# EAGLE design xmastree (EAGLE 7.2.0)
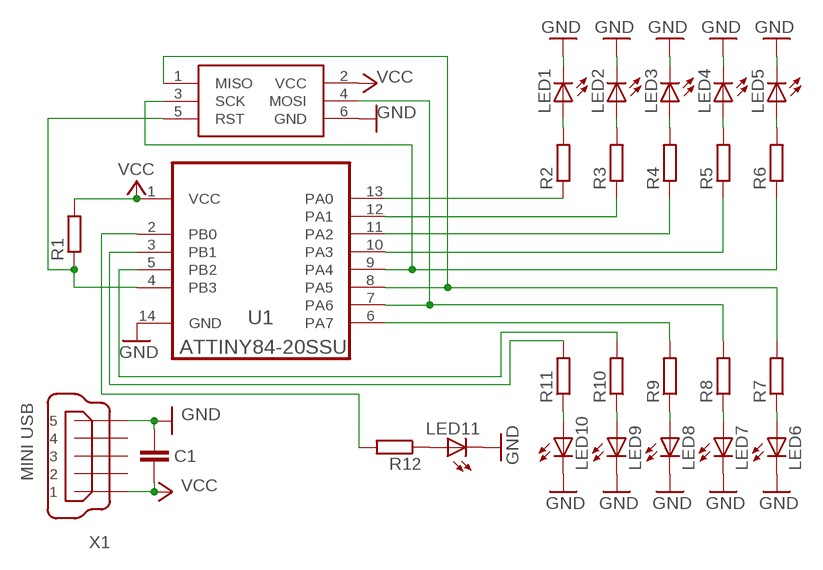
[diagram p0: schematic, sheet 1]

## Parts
C1  100nf  C-EUC1206  [C1206]
ISP1  AVRISP-6  [AVRISP]
LED1  LED3MM  [LED3MM]
LED2  LED3MM  [LED3MM]
LED3  LED3MM  [LED3MM]
LED4  LED3MM  [LED3MM]
LED5  LED3MM  [LED3MM]
LED6  LED3MM  [LED3MM]
LED7  LED3MM  [LED3MM]
LED8  LED3MM  [LED3MM]
LED9  LED3MM  [LED3MM]
LED10  LED3MM  [LED3MM]
LED11  LED5MM  [LED5MM]
R1  R-EU_R1206  [R1206]
R2  R-EU_R1206  [R1206]
R3  R-EU_R1206  [R1206]
R4  R-EU_R1206  [R1206]
R5  R-EU_R1206  [R1206]
R6  R-EU_R1206  [R1206]
R7  R-EU_R1206  [R1206]
R8  R-EU_R1206  [R1206]
R9  R-EU_R1206  [R1206]
R10  R-EU_R1206  [R1206]
R11  R-EU_R1206  [R1206]
R12  R-EU_R1206  [R1206]
U1  ATTINY84-20SSU  [SOIC127P600X175-14N]
X1  MINI USB  MINI-USB_SHIELD5P4-32005-400  [32005-400]

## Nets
GND: C1.1 ISP1.6(GND) LED1.K(C) LED2.K(C) LED3.K(C) LED4.K(C) LED5.K(C) LED6.K(C) LED7.K(C) LED8.K(C) LED9.K(C) LED10.K(C) LED11.K(C) U1.14(GND) X1.5
N$1: LED10.A R11.1
N$2: ISP1.5(RST) R1.1 U1.4(PB3)
N$3: LED7.A R8.1
N$4: LED8.A R9.1
N$5: ISP1.1(MISO) R7.2 U1.8(PA5)
N$6: ISP1.4(MOSI) R8.2 U1.7(PA6)
N$7: ISP1.3(SCK) R6.1 U1.9(PA4)
N$8: LED9.A R10.1
N$9: LED6.A R7.1
N$10: LED1.A R2.2
N$11: LED2.A R3.2
N$12: LED3.A R4.2
N$13: LED4.A R5.2
N$14: LED5.A R6.2
N$15: R12.2 U1.2(PB0)
N$16: R2.1 U1.13(PA0)
N$17: R3.1 U1.12(PA1)
N$18: R5.1 U1.10(PA3)
N$19: R4.1 U1.11(PA2)
N$21: R9.2 U1.6(PA7)
N$22: R10.2 U1.5(PB2)
N$23: R11.2 U1.3(PB1)
N$24: LED11.A R12.1
VCC: C1.2 ISP1.2(VCC) R1.2 U1.1(VCC) X1.1
Unconnected: X1.2 X1.3 X1.4 X1.M1(S1) X1.M2(S2) X1.M3(S3) X1.M4(S4)

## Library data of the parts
C1 = rcl:C-EU: CAPACITOR, European symbol
ISP1 = adafruit:AVRISP: AVR ISP HEADER Standard 6 pin header for AVR programming
LED1-LED11 = adafruit:LED: LED
R1-R12 = rcl:R-EU_: RESISTOR, European symbol
U1 = Atmel_By_element14_Batch_1-00:ATTINY84-20SSU: 8-bit Microcontroller with Bytes In-System Programmable Flash; MPN: ATTINY84-20SSU; OC_FARNELL: 1636955; OC_NEWARK: 03P2040; PACKAGE: SOIC-14; SUPPLIER: Atmel
X1 = con-cypressindustries:MINI-USB_SHIELD5P4-: MINI USB-B R/A W/O POST 5 pol. Source: www.cypressindustries.com; OC_FARNELL: unknown; OC_NEWARK: unknown

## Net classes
0 default: clearance 0.205 mm

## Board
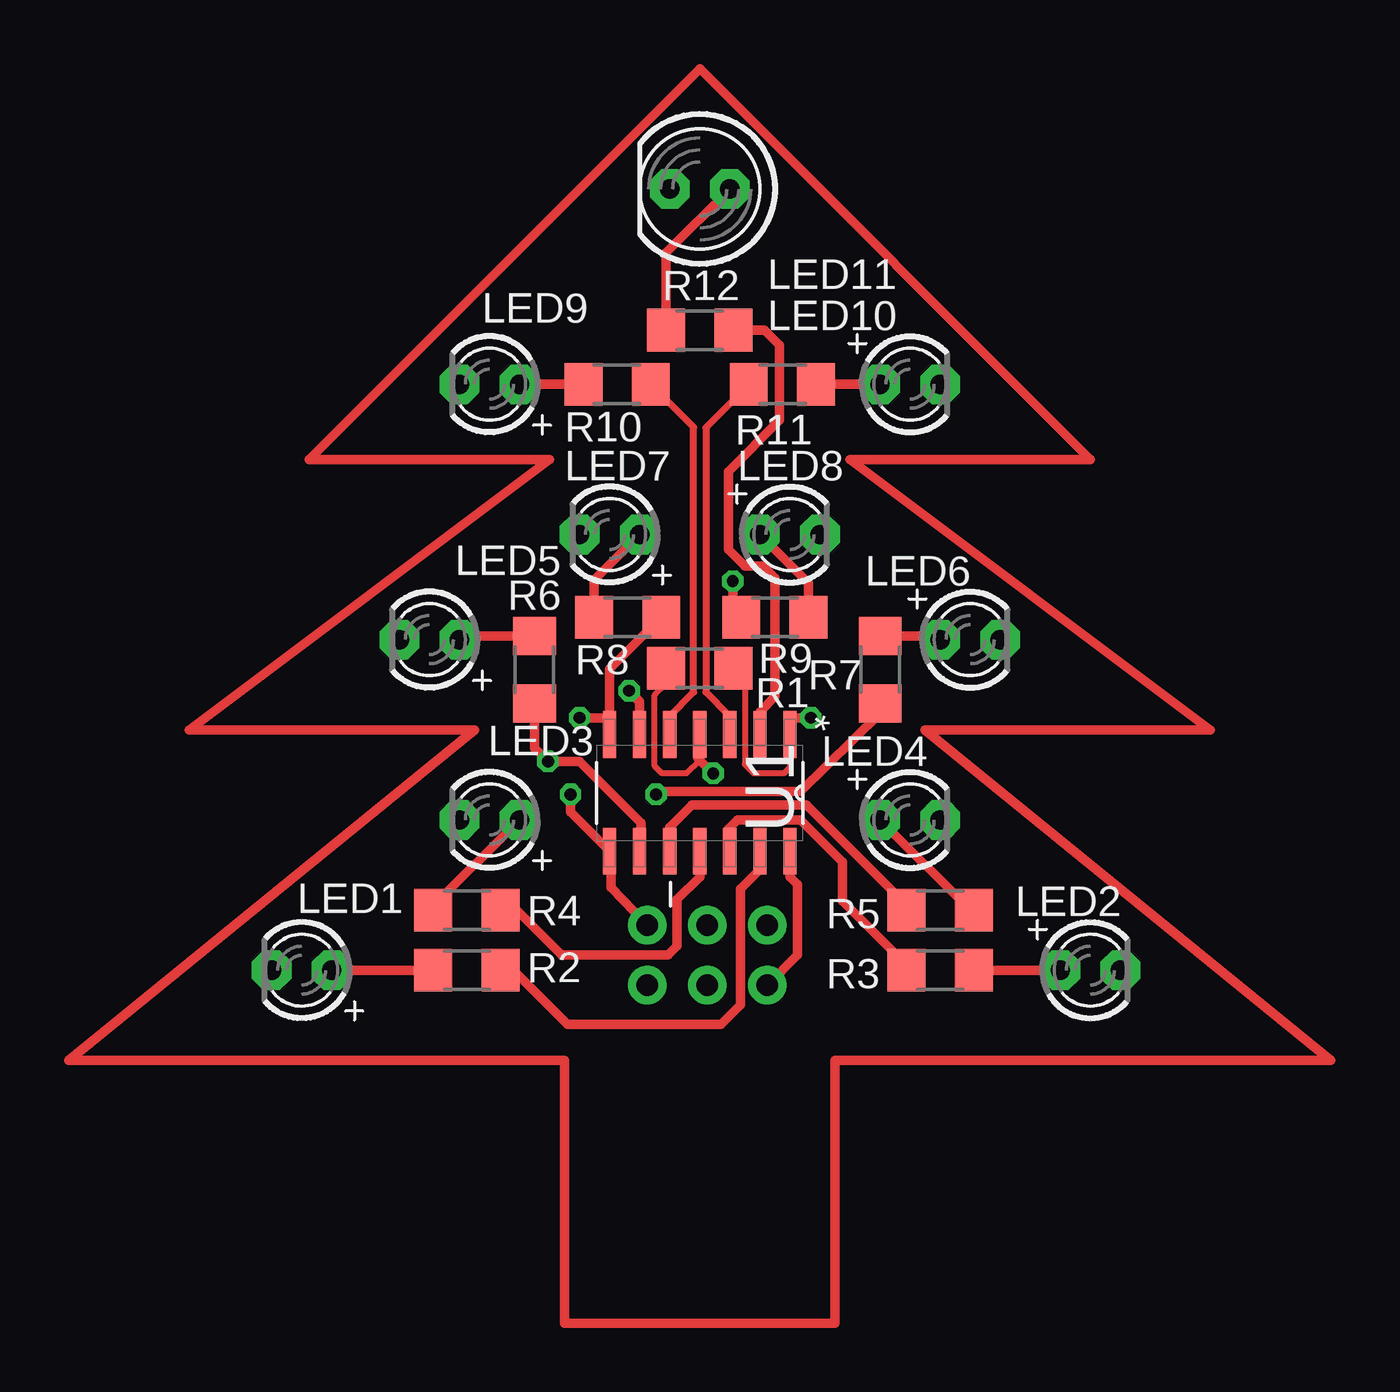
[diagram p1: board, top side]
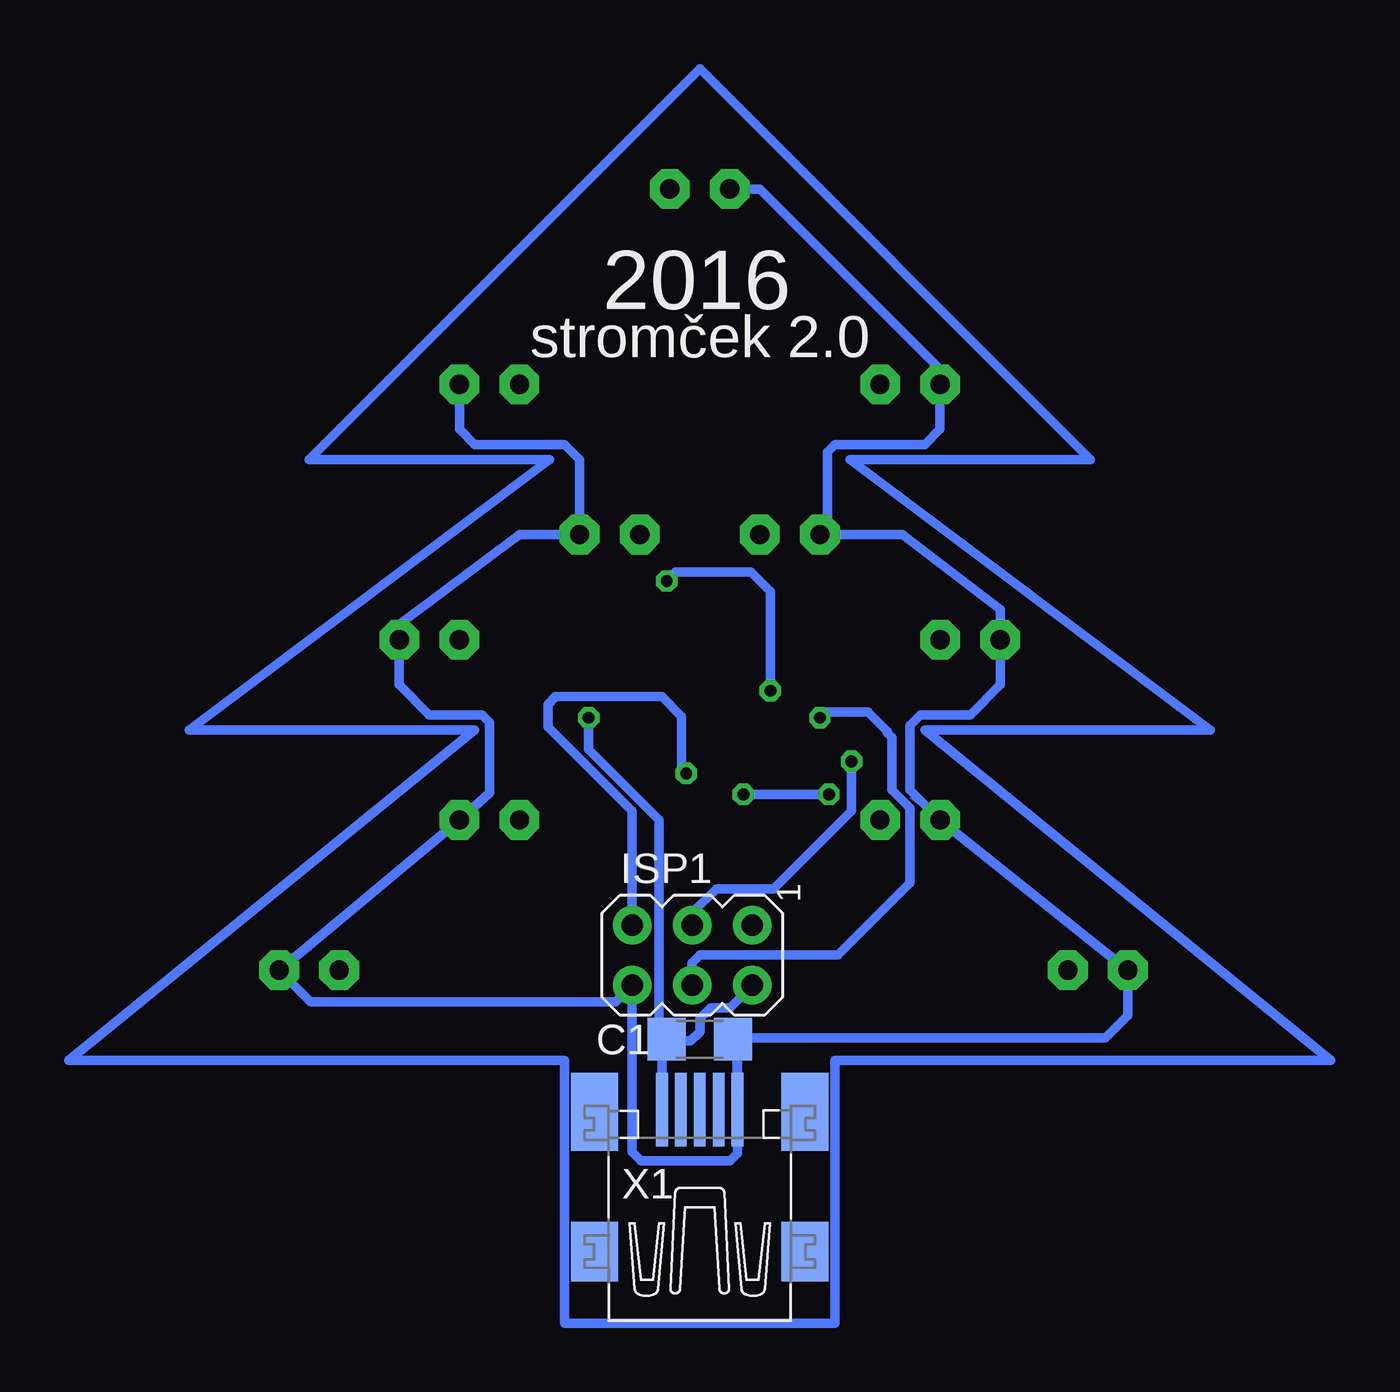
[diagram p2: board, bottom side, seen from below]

No outline drawn. Coordinates in mm, seen from the top.
Copper layers (1*16): Top 0.035mm / dielectric 1.5mm / Bottom 0.035mm
Design rules "default *": minimum track width 12mil, minimum drill 24mil, track to track 8mil, track to pad 8mil, pad to pad 8mil, via to via 8mil, smd to smd 8mil, copper to edge 40mil, drill to drill 8mil, minimum pad ring 10mil, minimum via ring 8mil, stop-mask expansion 4mil, vias tented up to drill 0mil, thermal gap 10mil

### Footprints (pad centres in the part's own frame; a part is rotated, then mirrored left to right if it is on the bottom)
C1206 = smd 1.6 x 1.8: 1 -1.4,0; 2 1.4,0
AVRISP = drill 0.9 pad 1.626: 1 -1.27,2.54; 2 1.27,2.54; 3 -1.27,0; 4 1.27,0; 5 -1.27,-2.54; 6 1.27,-2.54
LED3MM = drill 0.813 pad 1.676 octagon: A -1.27,0; K 1.27,0
LED5MM = drill 0.813 pad 1.676 octagon: A -1.27,0; K 1.27,0
R1206 = smd 1.6 x 1.803: 1 -1.422,0; 2 1.422,0
SOIC127P600X175-14N = smd 1.981 x 0.559: 1 -2.464,3.81; 2 -2.464,2.54; 3 -2.464,1.27; 4 -2.464,0; 5 -2.464,-1.27; 6 -2.464,-2.54; 7 -2.464,-3.81; 8 2.464,-3.81; 9 2.464,-2.54; 10 2.464,-1.27; 11 2.464,0; 12 2.464,1.27; 13 2.464,2.54; 14 2.464,3.81
32005-400 = smd 3.1 x 0.5: 1 3,1.6; 2 3,0.8; 3 3,0; 4 3,-0.8; 5 3,-1.6 | smd 2.5 x 2: M1 -3,-4.45; M2 -3,4.45 | smd 3.3 x 2: M3 2.9,4.45; M4 2.9,-4.45

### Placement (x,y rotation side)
C1  29.4,16.07 180 bottom
ISP1  29.72,19.62 270 bottom
LED1  12.57,18.99 180 top
LED2  45.91,18.99 0 top
LED3  20.51,25.34 180 top
LED4  38.29,25.34 0 top
LED5  17.97,32.96 180 top
LED6  40.83,32.96 0 top
LED7  25.59,37.4 180 top
LED8  33.21,37.4 0 top
LED9  20.51,43.75 180 top
LED10  38.29,43.75 0 top
LED11  29.4,52.01 180 top
R1  29.4,31.75 0 top
R2  19.56,18.99 180 top
R3  39.56,18.99 0 top
R4  19.56,21.53 180 top
R5  39.56,21.53 0 top
R6  22.42,31.69 90 top
R7  37.02,31.69 270 top
R8  26.35,33.91 0 top
R9  32.58,33.91 180 top
R10  25.91,43.75 0 top
R11  32.89,43.75 180 top
R12  29.4,46.04 0 top
U1  29.4,26.48 270 top
X1  29.4,10.1 90 bottom

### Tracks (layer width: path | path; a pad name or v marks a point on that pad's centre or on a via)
GND
  Top 0.406: U1.14 33.21,22.92 33.53,22.61 33.53,19.62 ISP1.6
  Bottom 0: 36.7,37.4 42.1,33.59 42.1,31.05 | 20.51,26.29 LED1.K
  Bottom 0.305: 27.76,15.98 C1.1 27.82,15.82 | 27.82,13.18 X1.5
  Bottom 0.406: LED11.K 26.86,52.01 19.24,44.39 LED9.K 19.24,41.85 19.88,41.21 23.69,41.21 24,40.89 24,37.72 LED7.K 20.83,37.4 16.7,34.23 LED5.K 16.7,31.05 17.97,29.78 20.07,29.78 20.51,29.34 20.51,26.61 LED3.K LED1.K 11.3,17.08 12.26,16.13 27.94,16.13 C1.1 | LED10.K 39.56,41.85 38.92,41.21 35.12,41.21 34.48,40.58 LED8.K 36.7,37.4 37.02,37.4 42.1,33.59 LED6.K 42.1,31.05 40.83,29.78 38.61,29.78 38.29,29.46 38.29,26.48 LED4.K LED2.K 45.85,17.65 32.96,17.65 ISP1.6 32.26,11.3 31.88,10.92 28.13,10.92 27.81,11.24 27.81,15.49 28,15.68 C1.1 | 27.82,13.18 27.82,15.88 C1.1
N$1
  Top 0.406: R11.1 LED10.A
N$2  (via drill 0.5)
  Top 0.254: 27.98,31.09 27.5,30.61 27.5,27.62 27.81,27.3 28.83,27.3 29.4,27.88 29.4,27.94 29.34,27.94
  Top 0.406: R1.1 27.98,31.09 | U1.4 29.34,28.88 29.34,27.94 v29.97,27.3
  Bottom 0.406: ISP1.5 32.26,25.72 35.81,29.27 35.81,30.23 35.5,30.54 30.99,30.54 30.16,29.72 30.16,27.5 v29.97,27.3
N$3
  Top 0.406: R8.1 24.93,35.47 LED7.A
N$4
  Top 0.406: R9.1 34,35.34 LED8.A
N$5  (via drill 0.5)
  Top 0.406: ISP1.1 27.11,20.95 25.65,22.48 25.65,23.95 U1.8 23.94,25.67 v23.94,26.42 | R7.2 37.02,29.84 33.66,26.54 27.69,26.54 v27.56,26.42
  Bottom 0.406: v27.56,26.42 v23.94,26.42
N$6  (via drill 0.5)
  Top 0.406: 25.59,29.64 25.59,31.73 R8.2 | v24.32,29.65 25.59,29.64 | 25.59,29.64 U1.7
  Bottom 0.406: ISP1.4 29.72,19.3 29.4,19.62 23.56,19.62 20.51,22.67 20.51,25.84 21.27,26.61 21.27,28.83 21.46,29.02 21.46,29.08 22.29,29.91 24.07,29.91 v24.32,29.65
N$7  (via drill 0.5)
  Top 0.406: U1.9 26.92,23.95 26.92,25.21 24.32,27.81 v22.99,27.81 22.42,28.38 R6.1 21.84,29.69
  Bottom 0.406: ISP1.3 29.72,21.4 28.7,22.42 26.29,22.42 22.99,25.72 v22.99,27.81
N$8
  Top 0.406: R10.1 LED9.A
N$9
  Top 0.406: R7.1 39.41,33.11 LED6.A
N$10
  Top 0.406: R2.2 LED1.A
N$11
  Top 0.406: LED2.A R3.2
N$12
  Top 0.406: R4.2 18.14,21.69 LED3.A
N$13
  Top 0.406: R5.2 40.83,21.53 LED4.A
N$14
  Top 0.406: R6.2 19.39,33.11 LED5.A
N$15
  Top 0.406: R12.2 32.13,46.04 32.77,45.4 32.77,42.23 30.61,40.07 30.61,36.77 31.3,36.07 32.07,36.07 32.58,35.56 32.58,30.54 31.94,29.91 U1.2
N$16
  Top 0.406: R2.1 21.53,18.99 23.81,16.7 30.29,16.7 31.11,17.53 31.11,22.42 31.88,23.18 31.88,23.95 U1.13
N$17
  Top 0.406: R3.1 38.14,19.2 35.43,21.91 35.43,23.56 33.66,25.34 30.99,25.34 30.61,24.96 30.61,24.08 U1.12
N$18
  Top 0.406: R5.1 38.14,21.74 33.91,25.97 29.08,25.97 28.13,25.02 U1.10
N$19
  Top 0.406: R4.1 21.65,21.53 23.56,19.62 28.07,19.62 28.45,20 28.45,21.97 29.4,22.92 U1.11
N$21  (via drill 0.5)
  Top 0.406: U1.6 26.86,30.35 v26.42,30.8 | v30.8,35.43 30.8,34.27 R9.2
  Bottom 0.406: v26.42,30.8 26.42,34.99 27.24,35.81 30.42,35.81 v30.8,35.43
N$22
  Top 0.305: U1.5 28.13,29.72 29.15,30.73 29.15,41.94 R10.2
N$23
  Top 0.305: R11.2 31.43,43.69 29.65,41.91 29.65,30.73 30.61,29.78 30.61,29.01 U1.3
N$24
  Top 0.406: R12.1 27.98,49.31 LED11.A
N$25
  Top 0.406: 23.69,4.06 35.12,4.06 35.12,15.18 56.07,15.18 38.92,29.15 50.99,29.15 35.75,40.58 45.91,40.58 29.4,57.09 12.89,40.58 23.05,40.58 7.81,29.15 19.88,29.15 2.73,15.18 23.69,15.18 23.69,4.06
S$3
  Bottom 0.406: 23.69,4.06 35.12,4.06 35.12,15.18 56.07,15.18 38.92,29.15 50.99,29.15 35.75,40.58 45.91,40.58 29.4,57.09 12.89,40.58 23.05,40.58 7.81,29.15 19.88,29.15 2.73,15.18 23.69,15.18 23.69,4.06
VCC  (via drill 0.5)
  Top 0.254: 31.37,31.27 31.37,31.11 31.3,31.05 31.3,27.69 31.69,27.3 32.96,27.3 33.21,27.56 U1.1
  Top 0.406: 31.37,31.27 R1.2 | v34.1,29.65 33.27,29.65 33.21,29.59 U1.1
  Bottom 0.406: X1.1 31,15.43 | 31,15.43 31,15.87 C1.2 30.74,16 29.78,16 29.4,16.38 29.4,16.95 28.96,17.4 28.13,17.4 ISP1.2 | v34.1,29.65 34.1,28.32 31.11,25.34 31.11,15.54 31,15.43

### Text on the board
bPlace: 2016 | stromček 2.0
